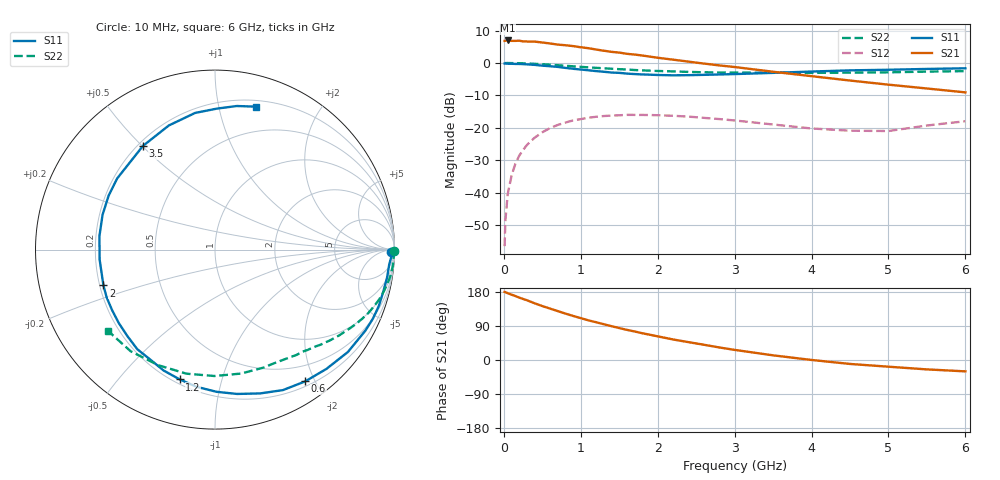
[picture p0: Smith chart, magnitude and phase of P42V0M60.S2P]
! SIEMENS Small Signal Semiconductors
! BFP182
! Si NPN RF Bipolar Junction Transistor in SOT143
! VCE = 2 V  IC = 0.6 mA
! Common Emitter S-Parameters:  March  1996
# GHz  S  MA  R  50
!  f  S11  S21  S12  S22
! GHz  MAG  ANG  MAG  ANG  MAG  ANG  MAG  ANG
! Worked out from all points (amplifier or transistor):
!   36 points, 10 MHz to 6 GHz, reference 50 ohm
!   highest |S21| = 6.9 dB at 50 MHz (marker M1)
!   |S21| within 3 dB of that: start of sweep to 1.255 GHz
!   unconditionally stable (mu >= 1): 2.855 GHz to end of sweep
!   at 250 MHz: K = 0.09, MSG = 16.7 dB, |S12| = -26.8 dB
!   at 1.4 GHz: K = 0.51, MSG = 9.8 dB, |S12| = -16.2 dB
!   at 6 GHz: K = 1.20, MAG = 1.8 dB, |S12| = -18.0 dB
!   S11 on the Smith chart (normalised r, x): 10 MHz: 62, -49; 600 MHz: 0.26, -1.87; 1.2 GHz: 0.22, -0.74; 2 GHz: 0.21, -0.15; 3.5 GHz: 0.22, +0.50; 6 GHz: 0.25, +1.29
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0.01  0.9804 -0.9  2.191 179.6  0.0015 85.3  0.9997 -0.3
0.02  0.9842 -2.1  2.203 179.2  0.0037 87.4  0.9949 -0.6
0.05  0.9743 -4.8  2.223 176.3  0.0095 88.5  0.9979 -1.7
0.1  0.9713 -9.2  2.19 172.5  0.0183 83.1  0.9946 -3.5
0.15  0.9664 -14.4  2.19 168.7  0.028 81.1  0.9944 -5.3
0.2  0.9653 -19.1  2.203 164.7  0.0372 77.6  0.9918 -7.0
0.4  0.9348 -37.6  2.135 149.7  0.0705 66.0  0.9701 -13.6
0.6  0.8898 -55.6  1.999 135.7  0.0992 54.3  0.9396 -19.8
0.8  0.8397 -72.6  1.877 122.5  0.1205 44.2  0.9058 -25.2
0.9  0.8136 -81.3  1.82 116.3  0.1302 39.2  0.8881 -27.8
1.1  0.7711 -97.7  1.689 104.6  0.1431 30.9  0.8555 -32.3
1.2  0.7494 -105.2  1.611 99.6  0.1482 26.4  0.8413 -34.6
1.4  0.7119 -120.0  1.484 89.2  0.1544 19.4  0.8148 -38.5
1.6  0.686 -135.3  1.383 79.5  0.1585 13.2  0.7927 -41.9
2  0.6529 -162.2  1.203 62.4  0.1565 2.8  0.7521 -48.8
2.2  0.6452 -175.0  1.124 54.2  0.1535 -1.9  0.7415 -52.4
2.8  0.6646 153.1  0.917 33.1  0.1366 -11.7  0.7128 -63.3
3.5  0.7035 124.8  0.732 12.3  0.1126 -16.4  0.7058 -78.1
4.5  0.7694 98.3  0.536 -10.4  0.0903 -5.4  0.7094 -103.0
5  0.7856 89.2  0.463 -17.7  0.0893 7.4  0.7175 -116.2
5.5  0.8091 81.4  0.404 -24.8  0.1086 13.1  0.7359 -129.7
6  0.8282 74.1  0.352 -30.0  0.1265 13.9  0.7483 -142.6
